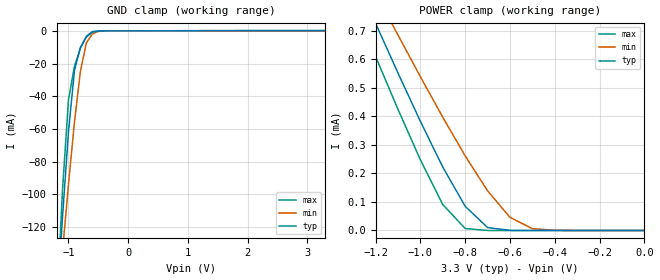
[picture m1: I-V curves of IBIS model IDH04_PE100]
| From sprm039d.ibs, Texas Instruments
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[Model]   IDH04_PE100
Model_type   Input
Polarity   Non-Inverting
| signals   A, Y
Vinl = 0.8V
Vinh = 2.0V
|   typ   min   max
C_comp   1.765p   1.745p   1.929p
|   typ   min   max
[Temperature Range]   25   -40   125
|   typ   min   max
[Voltage Range]   3.30V   3.00V   3.60V
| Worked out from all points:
|   GND clamp passes 1 mA (typ) near -0.61 V on its own axis
|   POWER clamp passes 1 mA (typ) near -1.35 V on its own axis
[GND_clamp]
|   Voltage   I(typ)   I(min)   I(max)
-3.3V     -1.513A    -1.145A    -1.96A
-1.2V     -171.8mA   -177.8mA   -171.3mA
-1.1V     -114.2mA   -135.1mA   -97.62mA
-1V       -61.87mA   -93.98mA   -42.24mA
-900mV    -24.33mA   -55.96mA   -21.71mA
-800mV    -10.06mA   -24.71mA   -10.67mA
-700mV    -3.783mA   -7.292mA   -3.241mA
-600mV    -786.5uA   -1.88mA    -447.9uA
-500mV    -112.8uA   -361.3uA   -87.29uA
-400mV    -39.84uA   -62.03uA   -56.2uA
3.3V      100.8uA    52.19uA    177.3uA
[POWER_clamp]
|   Voltage   I(typ)   I(min)   I(max)
-3.3V     4.588mA    4.102mA    4.731mA
-1.3V     903uA      983.5uA    798.1uA
-1.2V     725.8uA    833.2uA    609.3uA
-1.1V     551.6uA    684.6uA    424.5uA
-1V       382.2uA    538.7uA    247.4uA
-900mV    222.1uA    396.7uA    90.8uA
-800mV    84.67uA    261.3uA    6.783uA
-700mV    10.3uA     138.9uA    73.81nA
-600mV    329.7nA    46.05uA    888.2pA
-500mV    8.571nA    6.46uA     266.4pA
-400mV    444.1pA    466.5nA    222pA
0V        1pA        1pA        1pA
